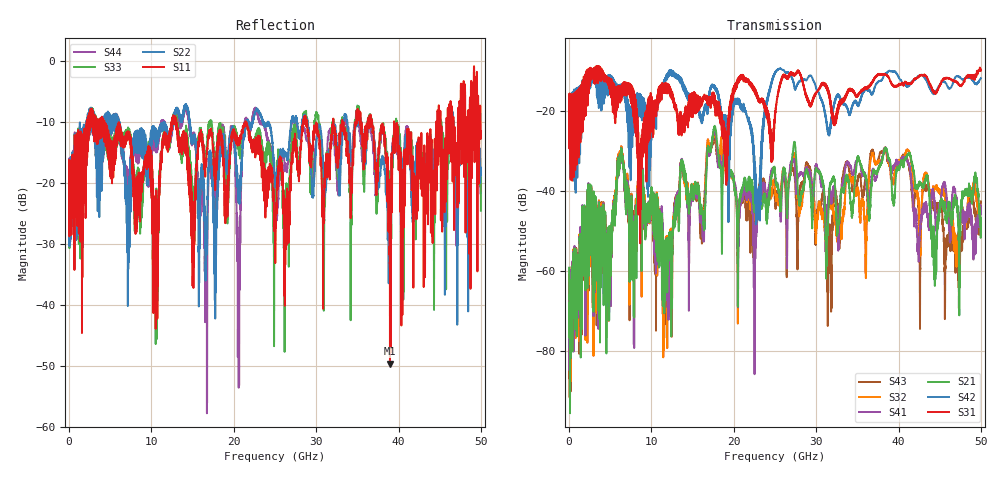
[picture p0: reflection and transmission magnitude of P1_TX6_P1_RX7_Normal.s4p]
!Keysight Technologies,N5225B,MY57041031,A.13.20.10
!Date: Friday, May 31, 2019 11:24:27
!Correction: S11(Full 4 Port(1,2,3,4))
!S12(Full 4 Port(1,2,3,4))
!S13(Full 4 Port(1,2,3,4))
!S14(Full 4 Port(1,2,3,4))
!S21(Full 4 Port(1,2,3,4))
!S22(Full 4 Port(1,2,3,4))
!S23(Full 4 Port(1,2,3,4))
!S24(Full 4 Port(1,2,3,4))
!S31(Full 4 Port(1,2,3,4))
!S32(Full 4 Port(1,2,3,4))
!S33(Full 4 Port(1,2,3,4))
!S34(Full 4 Port(1,2,3,4))
!S41(Full 4 Port(1,2,3,4))
!S42(Full 4 Port(1,2,3,4))
!S43(Full 4 Port(1,2,3,4))
!S44(Full 4 Port(1,2,3,4))
!S4P File: Measurements: <S11,S12,S13,S14>,
!<S21,S22,S23,S24>,
!<S31,S32,S33,S34>,
!<S41,S42,S43,S44>:
# Hz S  dB  R 50.0
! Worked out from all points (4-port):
!   5000 points, 10 MHz to 50 GHz, reference 50 ohm
!   strongest paths, dB at 10 MHz, 12.51 GHz, 25.01 GHz, 37.51 GHz, 50 GHz:
!     S31: -19.4, -15.5, -21.6, -10.8, -9.6
!     S42: -19.7, -9.9, -10.6, -12.7, -11.8
!     S21: -59.1, -60.0, -35.9, -34.8, -47.1
!     S41: -62.9, -57.2, -36.7, -34.9, -44.6
!     S32: -62.2, -66.9, -39.7, -32.5, -45.3
!     S43: -60.9, -62.7, -42.6, -32.4, -42.8
!   lowest |S11| = -49.7 dB at 38.96 GHz (marker M1), VSWR 1.01, Z = 50 + j0.327 ohm
!   |S11| at or under -10 dB: 4.286 GHz to 12.46 GHz (8.179 GHz wide, 97.7 % of centre); 13.02 GHz to 21.43 GHz (8.403 GHz wide, 48.8 % of centre); 21.46 GHz to 28.42 GHz (6.955 GHz wide, 27.9 % of centre)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
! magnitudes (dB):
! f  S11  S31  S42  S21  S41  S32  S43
! 10 MHz  -19.2  -19.4  -19.7  -59.1  -62.9  -62.2  -60.9
! 6.34 GHz  -13.7  -16.6  -14.2  -29.2  -29.2  -28.8  -28.7
! 11.68 GHz  -12.0  -13.5  -11.8  -52.2  -53.1  -53.8  -55.0
! 22.93 GHz  -13.1  -16.9  -39.6  -45.8  -45.8  -44.9  -42.1
! 25.27 GHz  -19.1  -16.9  -9.7  -38.3  -38.0  -41.0  -40.2
! 38.96 GHz  -49.7  -12.3  -10.0  -32.2  -33.2  -34.2  -33.4
! 50 GHz  -11.4  -9.6  -11.8  -47.1  -44.6  -45.3  -42.8
